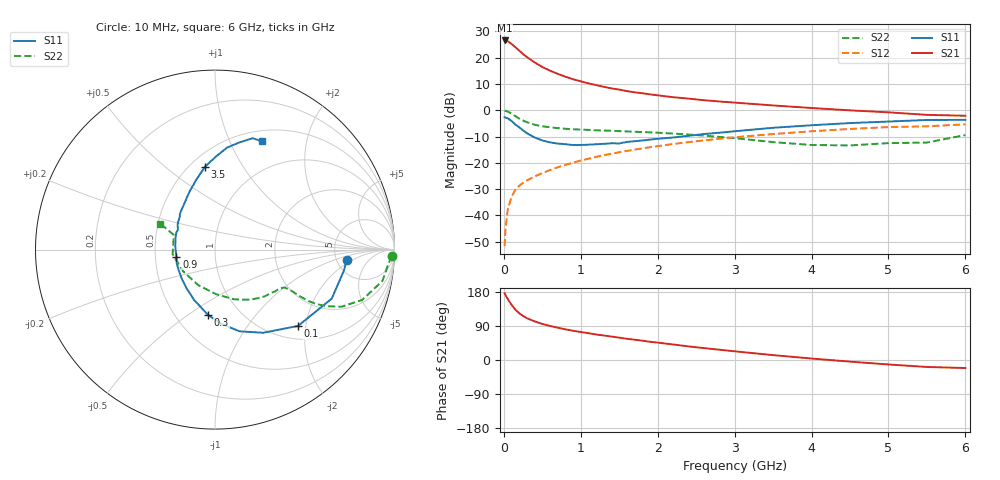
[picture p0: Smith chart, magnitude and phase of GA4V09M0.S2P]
! Infineon Technologies  Discrete & RF Semiconductors
! BF775
! Si NPN RF Bipolar Junction Transistor in SOT23
! VCE = 4 V  IC = 9 mA
! Common Emitter S-Parameters:  May  1996
# GHz  S  MA  R  50
!  f  S11  S21  S12  S22
! GHz  MAG  ANG  MAG  ANG  MAG  ANG  MAG  ANG
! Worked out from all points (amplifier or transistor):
!   36 points, 10 MHz to 6 GHz, reference 50 ohm
!   highest |S21| = 26.6 dB at 10 MHz (marker M1)
!   |S21| within 3 dB of that: start of sweep to 167 MHz
!   unconditionally stable (mu >= 1): 613.8 MHz to 3.127 GHz
!   at 250 MHz: K = 0.65, MSG = 24.5 dB, |S12| = -27.6 dB
!   at 1.4 GHz: K = 1.11, MAG = 10.4 dB, |S12| = -16.5 dB
!   at 6 GHz: K = 0.93, MSG = 1.6 dB, |S12| = -5.3 dB
!   S11 on the Smith chart (normalised r, x): 10 MHz: 6.16, -1.59; 100 MHz: 1.29, -1.81; 300 MHz: 0.71, -0.60; 900 MHz: 0.64, -0.05; 3.5 GHz: 0.59, +0.70; 6 GHz: 0.63, +1.33
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0.01  0.7361 -4.6  21.32 176.1  0.0026 89.6  0.9867 -2.1
0.02  0.7278 -9.2  21.31 172.0  0.0051 89.0  0.9713 -4.3
0.05  0.7054 -22.8  20.68 161.3  0.0127 78.3  0.9492 -10.6
0.1  0.6283 -42.6  18.33 145.9  0.0226 72.3  0.8662 -18.9
0.15  0.5356 -59.9  15.89 132.6  0.0307 65.4  0.7736 -24.3
0.2  0.4749 -73.4  13.68 123.4  0.0366 62.6  0.6968 -26.9
0.25  0.4154 -85.0  11.75 116.1  0.0417 61.3  0.6382 -28.3
0.3  0.3672 -95.9  10.29 110.2  0.0464 61.4  0.5939 -28.8
0.4  0.3037 -112.5  8.159 102.0  0.055 61.2  0.5315 -28.8
0.5  0.2675 -126.3  6.671 95.2  0.0638 62.4  0.4961 -28.4
0.6  0.2453 -139.3  5.676 89.9  0.073 63.2  0.4751 -28.3
0.7  0.2326 -150.3  4.949 85.2  0.0824 63.9  0.458 -28.4
0.9  0.2181 -169.8  3.902 77.2  0.1012 64.2  0.4361 -29.0
1.1  0.2218 175.7  3.259 70.7  0.1201 63.7  0.424 -31.0
1.3  0.2301 162.5  2.796 64.7  0.1401 62.8  0.4122 -33.3
1.6  0.25 146.5  2.319 56.0  0.1689 60.6  0.3968 -37.5
2.2  0.3036 125.0  1.775 41.0  0.2282 55.5  0.3607 -48.7
2.8  0.3741 109.5  1.473 27.2  0.2873 49.0  0.3116 -63.3
3.5  0.465 96.9  1.237 12.9  0.3534 40.4  0.2483 -88.7
4.5  0.5718 83.3  0.998 -4.3  0.4421 27.4  0.2147 -145.9
5.5  0.6552 71.3  0.819 -18.4  0.4954 12.7  0.2436 160.3
6  0.6573 66.4  0.788 -21.2  0.541 8.5  0.3381 154.7
